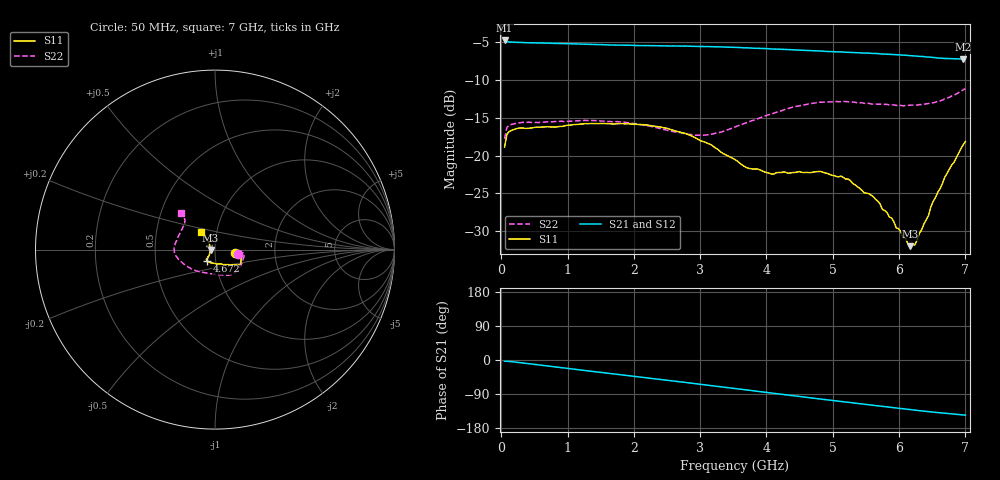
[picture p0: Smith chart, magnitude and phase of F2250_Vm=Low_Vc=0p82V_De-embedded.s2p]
! Integrated Device Technology
! Corporate Headquarters
! 6024 Silver Creek Valley Road
! San Jose, CA 95138  USA
! Phone:  1-408-284-8200
! Toll Free:  1-800-223-1366
! Webpage:  http://www.idt.com/
! Timing and RF Division
! 515 Groton Road, Suite 102
! Westford, MA 01886-6024
! Device:  F2250
! Description: Voltage Variable RF Attenuator
! Frequency:  50.0 -  6000.00 MHz
! Package:  3x3 mm Thin QFN Plastic Package: 16 pin
! Ports:  2 RF, 3 DC
!  Pin  1  = GND
!  Pin  2  = NC
!  Pin  3  = RF1  = Port 1
!  Pin  4  = NC
!  Pin  5  = GND
!  Pin  6  = GND
!  Pin  7  = GND
!  Pin  8  = GND
!  Pin  9  = NC
!  Pin 10  = RF2  = Port 2
!  Pin 11  = NC
!  Pin 12  = GND
!  Pin 13  = GND
!  Pin 14  = VCNTRL
!  Pin 15  = VDD
!  Pin 16  = VMODE
! Vcntrl:  0.820 Volts
! Vmode:  +0.000 Volts
! Vdd:  +3.30  Volts
! Current:  1.166 mA
! Data:  The device was measured on a the F2250 evaluation board which has
!  individual transmission lines to the RF pins.  Data was collected
!  using a calibrated network analyzer.  The evaluation board was
!  de-embedded using a TRL calibration technique.
!  The reference plane is the edge of the package pin.
! Misc:  SN 10
!  Action Tracker AT0258
! Date Measured:  2014-11-26
! Date:  2015-10-15  MJV
! Note:
!  Integrated Device Technology supplies this data as a sample of measured
!  data at the package pin for this product.  Your particular data for this
!  product may vary.
!  Data was taken at 25 degrees C.
!  Integrated Device Technology reserves the right to change this data at anytime.
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# GHz S dB R 50
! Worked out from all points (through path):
!   201 points, 50 MHz to 7 GHz, reference 50 ohm
!   highest |S21| = -4.74 dB at 50 MHz (marker M1); lowest = -7.2 dB at 6.965 GHz (marker M2)
!   group delay of S21, straight-line fit = 58.3 ps
!   lowest |S11| = -32.0 dB at 6.166 GHz (marker M3), VSWR 1.05, Z = 47.6 - j0.238 ohm
!   |S11| at or under -10 dB: start of sweep to end of sweep
!   |S22| runs from -17.8 to -11.1 dB; largest |S21 - S12| = 0.0016
!   S11 on the Smith chart (normalised r, x): 50 MHz: 1.25, -0.05; 4.672 GHz: 0.91, -0.12; 7 GHz: 0.84, +0.16
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0.05  -18.87 -10.2  -4.74 -3.3  -4.74 -3.3  -17.77 -9.8
0.08475  -17.17 -6.2  -4.89 -3.3  -4.90 -3.3  -16.26 -6.6
0.22375  -16.44 -7.0  -4.99 -5.8  -4.98 -5.8  -15.74 -9.7
1.2315  -15.81 -27.2  -5.23 -27.1  -5.24 -27.1  -15.34 -43.0
1.857  -15.80 -32.1  -5.37 -40.0  -5.37 -40.0  -15.57 -57.3
2.37825  -16.18 -34.2  -5.44 -50.7  -5.44 -50.7  -16.37 -70.1
3.0385  -18.13 -43.2  -5.53 -64.9  -5.53 -64.9  -17.31 -100.3
3.525  -20.53 -61.9  -5.66 -75.5  -5.65 -75.5  -16.21 -128.5
3.69875  -21.59 -72.4  -5.71 -79.3  -5.72 -79.3  -15.64 -137.1
4.081  -22.47 -96.9  -5.87 -87.5  -5.85 -87.5  -14.46 -154.0
4.67175  -22.26 -123.8  -6.09 -100.1  -6.08 -100.1  -13.08 -171.5
4.7065  -22.18 -125.0  -6.09 -100.8  -6.10 -100.8  -13.07 -172.2
5.22775  -23.10 -131.8  -6.30 -111.6  -6.30 -111.6  -12.85 176.0
5.471  -24.92 -132.2  -6.42 -116.6  -6.41 -116.6  -13.07 170.2
5.61  -25.45 -133.1  -6.46 -119.5  -6.45 -119.5  -13.19 166.6
5.85325  -28.15 -139.9  -6.58 -124.4  -6.59 -124.5  -13.28 160.2
5.888  -28.28 -141.8  -6.59 -125.2  -6.59 -125.2  -13.28 159.6
6.166  -32.01 -174.3  -6.75 -130.8  -6.75 -130.9  -13.34 150.4
6.2355  -31.86 167.7  -6.80 -132.2  -6.80 -132.3  -13.33 147.9
6.68725  -22.90 126.4  -7.14 -140.4  -7.12 -140.5  -12.47 135.0
6.96525  -18.59 129.0  -7.24 -145.0  -7.24 -145.0  -11.29 133.3
7  -18.14 129.0  -7.24 -145.5  -7.23 -145.6  -11.12 132.8
